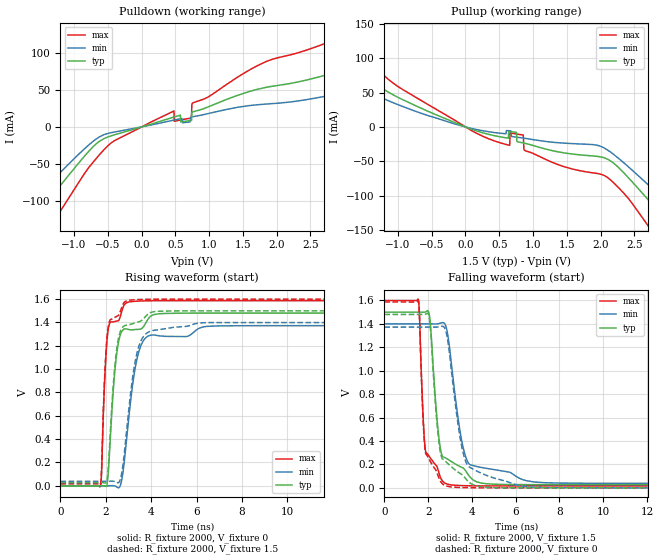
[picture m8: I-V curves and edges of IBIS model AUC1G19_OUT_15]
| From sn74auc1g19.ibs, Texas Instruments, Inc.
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[Model]   AUC1G19_OUT_15
Model_type  Output
Vref =   0
Rref =   2000
Cref =   15p
Vmeas =   0.75
| variable   typ   min   max
C_comp   6.24pF   1.95pF   19.03pF
| C_pullup   6.24pF   1.95pF   19.03pF
| C_pulldown   6.24pF   1.95pF   19.03pF
[Temperature Range]   40   100   -40
| Ambient temperature   25   85   -40
[Voltage range]   1.5   1.4   1.6
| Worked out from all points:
|   slope of the pulldown table from 0 to 0.225 V, typ, clamps not added: 36.6 ohm
|   slope of the pullup table from 0 to 0.225 V, typ, clamps not added: 29.5 ohm
|   rising waveform, R_fixture 2000, V_fixture 0: 20-80 % time 352ps typ, 536ps min, 218ps max; typ from 0 V to 1.48 V
|   falling waveform, R_fixture 2000, V_fixture 1.5: 20-80 % time 399ps typ, 622ps min, 232ps max; typ from 1.5 V to 0.027 V
|   rising waveform, R_fixture 2000, V_fixture 1.5: 20-80 % time 346ps typ, 529ps min, 214ps max; typ from 0.027 V to 1.5 V
|   falling waveform, R_fixture 2000, V_fixture 0: 20-80 % time 400ps typ, 629ps min, 230ps max; typ from 1.48 V to 0 V
[Pulldown]
| AUC1G19_OUT_15
|   Voltage   I(typ)   I(min)   I(max)
-3.6V     -346.8mA   -288.9mA   -430.8mA
-2.11V    -181.5mA   -146.5mA   -236.6mA
-1.795V   -146.1mA   -116.7mA   -194.8mA
-1.4V     -101.3mA   -79.49mA   -141.2mA
-400mV    -10.58mA   -6.84mA    -18.55mA
480mV     13.33mA    9.224mA    21.44mA
485mV     13.46mA    9.315mA    7.619mA
735mV     8.725mA    13.39mA    12.06mA
755mV     20.22mA    13.69mA    32.02mA
1.69V     50.07mA    29.62mA    81.22mA
3.345V    86.22mA    50.09mA    134.5mA
7.2V      80.6mA     45.5mA     140.4mA
[Pullup]
| AUC1G19_OUT_15
|   Voltage   I(typ)   I(min)   I(max)
-3.6V     253.3mA    195.3mA    303.6mA
-2.875V   187mA      147.7mA    233.1mA
-2.45V    149.4mA    116mA      191.6mA
-1.91V    104.2mA    79.13mA    139.3mA
100mV     -3.652mA   -2.395mA   -5.808mA
650mV     -6.722mA   -5.654mA   -26.6mA
855mV     -23.22mA   -16.17mA   -11.7mA
885mV     -23.88mA   -16.62mA   -34.51mA
2.105V    -46.98mA   -33.69mA   -73.66mA
2.765V    -112.5mA   -89.61mA   -152mA
3.365V    -180.2mA   -145.9mA   -234.3mA
7.2V      -612.6mA   -517.4mA   -745.9mA
[Ramp]
| AUC1G19_OUT_15
| variable   typ   min   max
dV/dt_r   0.89/3.53E-10   0.83/5.40E-10   0.96/2.19E-10
dV/dt_f   0.89/4.01E-10   0.82/6.28E-10   0.96/2.32E-10
R_load = 2000
[Rising Waveform]
| AUC1G19_OUT_15
R_fixture =   2000
C_fixture =   0
L_fixture =   0
V_fixture =   0
V_fixture_min = 0
V_fixture_max = 0
|   Time   V(typ)   V(min)   V(max)
0s        7.019nV    26.23nV    876.1pV
1.76ns    198.4uV    -1.346uV   -1.877mV
1.97ns    -4.338mV   -42.21uV   993.3mV
2.1ns     93.99mV    306.9uV    1.335V
2.49ns    1.148V     -10.15mV   1.412V
2.71ns    1.325V     60.79mV    1.5V
2.975ns   1.341V     515.4mV    1.574V
3.41ns    1.341V     1.119V     1.583V
3.975ns   1.454V     1.291V     1.586V
24.99ns   1.481V     1.373V     1.587V
[Falling Waveform]
| AUC1G19_OUT_15
R_fixture =   2000
C_fixture =   0
L_fixture =   0
V_fixture =   1.5
V_fixture_min = 1.4
V_fixture_max = 1.6
|   Time   V(typ)   V(min)   V(max)
0s        1.5V       1.4V       1.6V
1.55ns    1.5V       1.4V       1.611V
1.82ns    1.499V     1.4V       435mV
2.02ns    1.501V     1.4V       276.8mV
2.5ns     413.2mV    1.403V     123.2mV
2.865ns   248.1mV    1.338V     32.31mV
3.49ns    178.9mV    445.9mV    19.67mV
3.93ns    88.61mV    196.2mV    17.72mV
7.365ns   27.4mV     43.53mV    16.46mV
24.99ns   27.2mV     38.78mV    16.41mV
[Rising Waveform]
| AUC1G19_OUT_15
R_fixture =   2000
C_fixture =   0
L_fixture =   0
V_fixture =   1.5
V_fixture_min = 1.4
V_fixture_max = 1.6
|   Time   V(typ)   V(min)   V(max)
0s        27.17mV    38.78mV    16.4mV
1.755ns   27.34mV    38.78mV    12.63mV
1.97ns    24.02mV    38.74mV    1.021V
2.095ns   122.3mV    39.05mV    1.35V
2.47ns    1.156V     32.18mV    1.451V
2.68ns    1.341V     88.68mV    1.519V
2.91ns    1.377V     462.4mV    1.585V
3.39ns    1.403V     1.152V     1.596V
4.055ns   1.49V      1.331V     1.599V
24.99ns   1.5V       1.4V       1.6V
[Falling Waveform]
| AUC1G19_OUT_15
R_fixture =   2000
C_fixture =   0
L_fixture =   0
V_fixture =   0
V_fixture_min = 0
V_fixture_max = 0
|   Time   V(typ)   V(min)   V(max)
0s        1.481V     1.373V     1.587V
1.55ns    1.481V     1.373V     1.597V
1.815ns   1.48V      1.373V     425.6mV
2.015ns   1.48V      1.373V     254mV
2.49ns    393.1mV    1.375V     85.6mV
2.83ns    219.7mV    1.324V     15.93mV
3.385ns   132.5mV    515.8mV    3.785mV
3.685ns   85.3mV     241.4mV    2.004mV
5.01ns    2.926mV    83.42mV    227.2uV
24.99ns   23.8uV     2.176uV    9.951uV
